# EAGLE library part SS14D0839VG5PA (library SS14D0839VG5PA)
Slide Switches Source: Datasheet
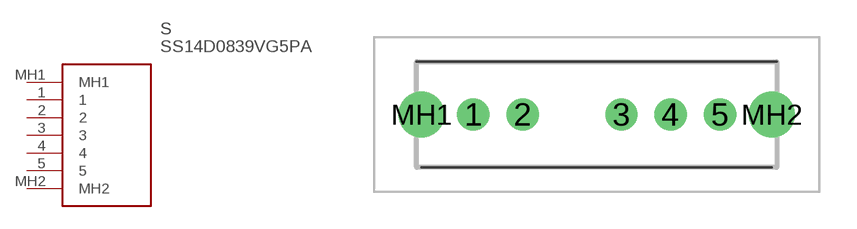
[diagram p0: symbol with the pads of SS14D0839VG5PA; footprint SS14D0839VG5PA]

Designator prefix S

## SS14D0839VG5PA (Description: Slide Switches; Height: 6.7mm; Manufacturer_Name: C & K COMPONENTS; Manufacturer_Part_Number: SS14D0839VG5PA; Mouser_Part_Number: 611-SS-14D0839-VG5PA; Mouser_Price-Stock: https://www.mouser.co.uk/ProductDetail/CK/SS14D0839VG5PA?qs=MLItCLRbWswItCuu%252BMrLYg%3D%3D)  [SS14D0839VG5PA]
1  1
2  2
3  3
4  4
5  5
MH1  MH1
MH2  MH2

## Footprint SS14D0839VG5PA (pad centres in mm)
SS14D0839VG5PA-4
drill 0.8 pad 1.3: 1 0,0; 2 2,0; 3 6,0; 4 8,0; 5 10,0
drill 1.25 pad 1.875: MH1 -2.1,0; MH2 12.1,0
